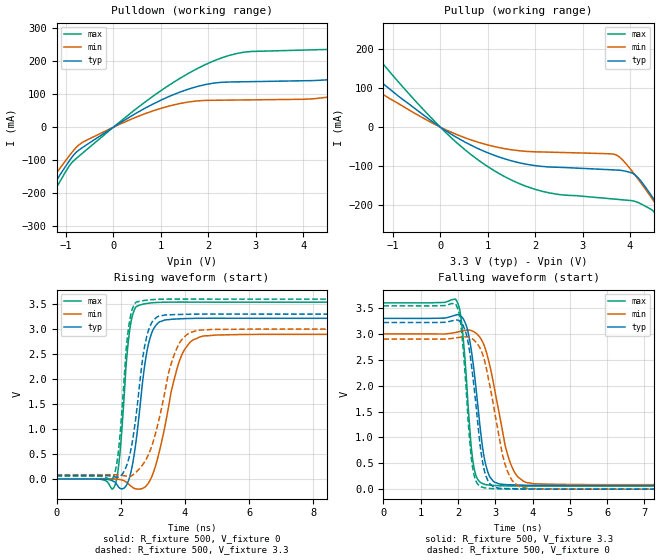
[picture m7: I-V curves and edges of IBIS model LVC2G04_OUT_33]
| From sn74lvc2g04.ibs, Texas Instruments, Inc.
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[Model]   LVC2G04_OUT_33
Model_type  Output
Vref =   0
Rref =   500
Cref =   50p
Vmeas =   1.5
| variable   typ   min   max
C_comp   9.43pF   5.86pF   12.63pF
| C_pullup   9.92pF   5.86pF   11.98pF
| C_pulldown   8.95pF   6.08pF   12.63pF
[Temperature Range]   40   100   -40
| Ambient temperature   25   85   -40
[Voltage range]   3.3   3   3.6
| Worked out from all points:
|   slope of the pulldown table from 0 to 0.495 V, typ, clamps not added: 11.3 ohm
|   slope of the pullup table from 0 to 0.495 V, typ, clamps not added: 13.6 ohm
|   rising waveform, R_fixture 500, V_fixture 0: 20-80 % time 369ps typ, 590ps min, 249ps max; typ from 0 V to 3.22 V
|   falling waveform, R_fixture 500, V_fixture 3.3: 20-80 % time 315ps typ, 487ps min, 220ps max; typ from 3.3 V to 0.069 V
|   rising waveform, R_fixture 500, V_fixture 3.3: 20-80 % time 391ps typ, 655ps min, 257ps max; typ from 0.069 V to 3.3 V
|   falling waveform, R_fixture 500, V_fixture 0: 20-80 % time 304ps typ, 459ps min, 218ps max; typ from 3.22 V to 0 V
[Pulldown]
| LVC2G04_OUT_33
|   Voltage   I(typ)   I(min)   I(max)
-5.5V     -1.112A    -993.8mA   -1.259A
-2.645V   -490.3mA   -433.2mA   -553.8mA
-1.49V    -226.9mA   -197.7mA   -257.3mA
-540mV    -51.04mA   -37.69mA   -65.27mA
1.025V    83.38mA    58mA       112.9mA
2.285V    136mA      81.66mA    210.1mA
4.75V     148.7mA    96.8mA     237.9mA
6.98V     278.7mA    201.6mA    396.3mA
7.35V     308.5mA    129.4mA    437mA
7.84V     330.1mA    92.52mA    494.2mA
8.75V     170.8mA    93.27mA    500.6mA
11V       160mA      96.49mA    276.8mA
[Pullup]
| LVC2G04_OUT_33
|   Voltage   I(typ)   I(min)   I(max)
-5.5V     609.5mA    479.2mA    854.2mA
-3.13V    322.5mA    249.3mA    458mA
-2.385V   237.2mA    181.8mA    339.2mA
-1.845V   177.9mA    135.2mA    255.8mA
-130mV    10.97mA    8.025mA    16.16mA
1.04V     -67.46mA   -46.7mA    -103.9mA
2.145V    -100.4mA   -63.42mA   -163.8mA
3.71V     -109.5mA   -71.26mA   -184.2mA
4.15V     -126.7mA   -129.5mA   -191.6mA
4.765V    -233mA     -235.6mA   -263.4mA
4.95V     -268.4mA   -268.9mA   -301.3mA
11V       -1.523A    -1.428A    -1.684A
[Ramp]
| LVC2G04_OUT_33
| variable   typ   min   max
dV/dt_r   2.05/4.03E-10   1.86/6.48E-10   2.24/2.73E-10
dV/dt_f   1.98/3.32E-10   1.79/5.16E-10   2.17/2.35E-10
R_load = 500
[Rising Waveform]
| LVC2G04_OUT_33
R_fixture =   500
C_fixture =   0
L_fixture =   0
V_fixture =   0
V_fixture_min = 0
V_fixture_max = 0
|   Time   V(typ)   V(min)   V(max)
0s        141.8pV    4.978nV    2.659nV
1.805ns   -55.84mV   -202.6uV   -146.8mV
1.965ns   -180.8mV   -10.35mV   451.8mV
2.3ns     92.7mV     -131.5mV   3.069V
2.715ns   2.125V     -176.2mV   3.502V
2.895ns   2.781V     -45.39mV   3.521V
3.16ns    3.123V     441.4mV    3.534V
3.835ns   3.206V     2.377V     3.541V
4.545ns   3.217V     2.858V     3.54V
24.99ns   3.216V     2.894V     3.539V
[Falling Waveform]
| LVC2G04_OUT_33
R_fixture =   500
C_fixture =   0
L_fixture =   0
V_fixture =   3.3
V_fixture_min = 3
V_fixture_max = 3.6
|   Time   V(typ)   V(min)   V(max)
0s        3.3V       3V         3.6V
1.96ns    3.369V     3.032V     3.644V
2.12ns    3.315V     3.06V      3.063V
2.26ns    3.07V      3.072V     1.744V
2.405ns   2.438V     3.049V     521.4mV
2.74ns    484.1mV    2.697V     88.21mV
2.955ns   148.8mV    2.036V     71.72mV
3.355ns   85.07mV    610.2mV    61.84mV
3.865ns   74.83mV    122.6mV    58.79mV
24.99ns   69.39mV    85.93mV    58.96mV
[Rising Waveform]
| LVC2G04_OUT_33
R_fixture =   500
C_fixture =   0
L_fixture =   0
V_fixture =   3.3
V_fixture_min = 3
V_fixture_max = 3.6
|   Time   V(typ)   V(min)   V(max)
0s        69.35mV    85.87mV    58.92mV
1.76ns    50.02mV    86.53mV    27.39mV
1.94ns    40.41mV    81.18mV    631.8mV
2.25ns    406.9mV    52.6mV     3.054V
2.555ns   1.704V     187.7mV    3.553V
2.75ns    2.675V     349.9mV    3.575V
3ns       3.167V     725.1mV    3.591V
3.695ns   3.291V     2.538V     3.601V
4.4ns     3.3V       2.974V     3.601V
24.99ns   3.3V       3V         3.6V
[Falling Waveform]
| LVC2G04_OUT_33
R_fixture =   500
C_fixture =   0
L_fixture =   0
V_fixture =   0
V_fixture_min = 0
V_fixture_max = 0
|   Time   V(typ)   V(min)   V(max)
0s        3.22V      2.9V       3.542V
1.945ns   3.267V     2.923V     3.568V
2.1ns     3.207V     2.94V      3.027V
2.245ns   2.938V     2.941V     1.646V
2.39ns    2.224V     2.902V     429.7mV
2.595ns   840.1mV    2.719V     56.97mV
2.72ns    324.6mV    2.461V     24.7mV
3.26ns    11.49mV    487.6mV    3.397mV
3.74ns    4.94mV     27.75mV    182.5uV
24.99ns   35.28uV    45.58uV    36.31uV
